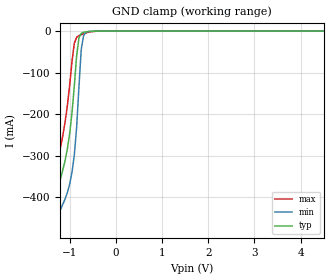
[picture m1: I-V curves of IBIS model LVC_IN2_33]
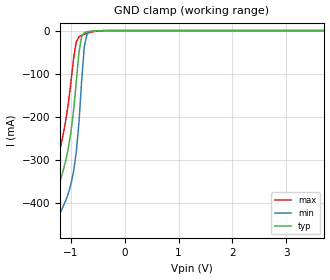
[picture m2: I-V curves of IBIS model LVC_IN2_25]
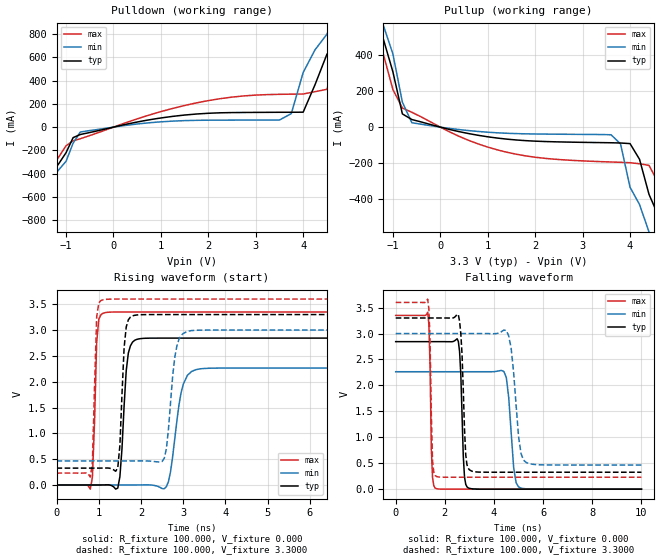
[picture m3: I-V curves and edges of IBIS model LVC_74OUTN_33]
| Philips Semiconductors Inc.
| Logic Products Group
| IBIS model of 74LVC74A
| DUAL D-TYPE FLIP-FLOP WITH SET AND RESET; POSITIVE-EDGE TRIGGER
|[Packages]:
|[Package1]: SO 14-pin (D) Package ;
|[Package2]: SSOP 14-Pin Packages ;
|[Package3]: TSSOP 14-pin (PW) Package ;
[IBIS Ver]   3.2
[File Name]   lvc74a.ibs
[File Rev]   1.3
[Date]   26-Nov-2002
[Source]   File created from simulations by LPG
   Philips Semiconductors Nijmegen
[Notes]   V1.3   Ibis model.
| Remark:
| The Power Clamp curves have been omitted since there is no power clamp diode.
| Revision History
| Version Date   Author/ Description
|   Editor
| 1.0   1999   Initial Version
| 1.1   October, 2001 RM   Revised for Ibis 3.2:
|   Model Spec and Model Selector added
| 1.2   November 2001 RM   Monotonous Curves
| 1.3   November 2002 RM   Revised: Power Clamp curves omitted, constant
|   end points for Ground Clamp and V/t curves.
[Disclaimer]
   (C) Copyright 2002 Philips Semiconductors
   All rights reserved
   Philips Semiconductors warrants and represents that the IBIS model
   identified herein is owned by Philips Semiconductors (PHILIPS). The
   model provided is not warranted as fully representing all of the
   operating characteristics and specifications of the semiconductor
   products to which the model relates.  Moreover, unless there is a
   signed, written agreement to the contrary, this IBIS model is
   furnished on an "as is" basis without support or warranty of any
   kind, either expressed or implied, regarding the use thereof, and
   PHILIPS specifically disclaims all implied warranties of
   merchantability and fitness of the model for any purpose.
   PHILIPS does not assume any liability arising out of the application
   or use of this IBIS model including infringement of patents and
   copyrights, nor does PHILIPS convey any license under its patents and
   copyrights or the rights of others.
   PHILIPS provides IBIS models as a service to our customers. You and
   your company shall not distribute, convey, sell, or give these models
   to anyone else without receiving prior written permission from
   PHILIPS.
   PHILIPS reserves the right to make changes without notice to these
   IBIS models to improve reliability, function, or design.
   Please be aware that your receipt and subsequent use of the IBIS
   information provided shall serve as acceptance of the terms and
   conditions of this agreement.  If you do not accept these terms,
   you should return or destroy the IBIS models and any other
   accompanying information immediately.
| to specify a consistent format that can be parsed by software, allowing
| simulation vendors to derive models compatible with their own products.
| One goal of this template is to represent the current state of IBIS data,
| while allowing a growth path to more complex models / methods (when deemed
| appropriate).  This would be accomplished by a revision of the base
| template, and possibly the addition of new keywords or categories.
| Another goal of this template is to ensure that it is simple enough for
| semiconductor vendors and customers to use and modify, while ensuring that
| it is rigid enough for simulation vendors to write reliable parsers.
| Finally, this template is meant to contain a complete description of the I/O
| elements on an entire component.  Consequently, several models will need to
| be defined in each file, as well as a table that equates the appropriate
| buffer to the correct pin and signal name.
| Version 3.2 of this electronic template was finalized by an industry-wide
| group of experts representing various companies and interests.  Regular
| "EIA IBIS Open Forum" meetings were held to accomplish this task.
| Commitment to Backward Compatibility.  Version 1.0 is the first valid IBIS
| ASCII file format.  It represents the minimum amount of I/O buffer
| information required to create an accurate IBIS model of common CMOS and
| bipolar I/O structures.  Future revisions of the ASCII file will add items
| considered to be "enhancements" to Version 1.0 to allow accurate modeling
| of new, or other I/O buffer structures.  Consequently, all future revisions
| will be considered supersets of Version 1.0, allowing backward
| compatibility.  In addition, as modeling platforms develop support for
| revisions of the IBIS ASCII template, all previous revisions of the template
| must also be supported.
| Version 1.1 update.  The file "ver1_1.ibs" is conceptually the same as the
| 1.0 version of the IBIS ASCII format (ver1_0.ibs).  However, various
| comments have been added for further clarification.
| Version 2.0 update.  The file "ver2_0.ibs" maintains backward compatibility
| with Versions 1.0 and 1.1.  All new keywords and elements added in Version
| 2.0 are optional.  A complete list of changes to the specification is in the
| IBIS Version 2.0 Release Notes document ("ver2_0.rn").
| Version 2.1 update.  The file "ver2_1.ibs" contains clarification text
| changes, corrections, and two additional waveform parameters beyond
| Version 2.0.
| Version 3.0 update.  The file "ver3_0.ibs" adds a number of new keywords
| and functionality.  A complete list of functions can be found on eda.org
| under /pub/ibis/birds/birddir.txt showing the approved Buffer Issue
| Resolution Documents (BIRDs) that have been approved for Version 3.0.
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[Component]   74LVC74A_1
[Manufacturer]   Philips Semiconductors Inc.
[Package]
|   typ   min   max
R_pkg   4.54E-02   4.18E-02   5.01E-02
L_pkg   2.31E-09   1.63E-09   3.26E-09
C_pkg   0.565E-12  0.437E-12  0.736E-12
[Pin] signal_name   model_name   R_pin   L_pin   C_pin
   1   1RD#   lvc_in2 4.18E-02 3.26E-09 0.675E-12
   2   1D   lvc_in2 5.01E-02 2.30E-09 0.574E-12
   3   1CP   lvc_in2 4.52E-02 1.71E-09 0.467E-12
   4   1SD#   lvc_in2 4.38E-02 1.63E-09 0.437E-12
   5   1Q   lvc_74outn 4.52E-02 1.71E-09 0.465E-12
   6   1QBAR#   lvc_74outi 5.01E-02 2.30E-09 0.573E-12
   7   GND   GND 4.18E-02 3.26E-09 0.736E-12
   8   2QBAR#   lvc_74outi 4.18E-02 3.26E-09 0.736E-12
   9   2Q   lvc_74outn 5.01E-02 2.30E-09 0.573E-12
   10   2SD#   lvc_in2 4.52E-02 1.71E-09 0.465E-12
   11   2CP   lvc_in2 4.38E-02 1.63E-09 0.437E-12
   12   2D   lvc_in2 4.52E-02 1.71E-09 0.467E-12
   13   2RD#   lvc_in2 5.01E-02 2.30E-09 0.574E-12
   14   VCC   POWER 4.18E-02 3.26E-09 0.736E-12
|   Info for  SSOP 14-Pin Packages
[Component]   74LVC74A_2
[Manufacturer]   Philips Semiconductors Inc.
[Package]
|   typ   min   max
R_pkg   18.10E-03   15.70E-03   19.10E-03
L_pkg   2.12E-09   1.76E-09   2.65E-09
C_pkg   0.59E-12   0.55E-12   0.64E-12
[Pin] signal_name   model_name   R_pin   L_pin   C_pin
   1   1RD#   lvc_in2 19.10E-03 2.65E-09 0.58E-12
   2   1D   lvc_in2 17.70E-03 2.07E-09 0.64E-12
   3   1CP   lvc_in2 18.70E-03 1.82E-09 0.57E-12
   4   1SD#   lvc_in2 15.70E-03 1.76E-09 0.55E-12
   5   1Q   lvc_74outn 18.70E-03 1.82E-09 0.57E-12
   6   1QBAR#   lvc_74outi 17.70E-03 2.07E-09 0.63E-12
   7   GND   GND 19.10E-03 2.65E-09 0.60E-12
   8   2QBAR#   lvc_74outi 19.10E-03 2.65E-09 0.60E-12
   9   2Q   lvc_74outn 17.80E-03 2.07E-09 0.64E-12
   10   2SD#   lvc_in2 18.70E-03 1.82E-09 0.57E-12
   11   2CP   lvc_in2 15.70E-03 1.76E-09 0.55E-12
   12   2D   lvc_in2 18.70E-03 1.82E-09 0.57E-12
   13   2RD#   lvc_in2 17.80E-03 2.07E-09 0.64E-12
   14   VCC   POWER 19.10E-03 2.65E-09 0.60E-12
|   Info for  TSSOP 14-pin (PW) Package
[Component]   74LVC74A_3
[Manufacturer]   Philips Semiconductors Inc.
[Package]
|   typ   min   max
R_pkg   3.44E-02   2.80E-02   4.33E-02
L_pkg   1.83E-09   1.36E-09   2.32E-09
C_pkg   0.380E-12  0.302E-12  0.442E-12
[Pin] signal_name   model_name   R_pin   L_pin   C_pin
   1   1RD#   lvc_in2 3.46E-02 2.32E-09 0.423E-12
   2   1D   lvc_in2 4.33E-02 2.04E-09 0.441E-12
   3   1CP   lvc_in2 2.80E-02 1.36E-09 0.307E-12
   4   1SD#   lvc_in2 2.88E-02 1.38E-09 0.302E-12
   5   1Q   lvc_74outn 2.80E-02 1.36E-09 0.308E-12
   6   1QBAR#   lvc_74outi 4.33E-02 2.04E-09 0.441E-12
   7   GND   GND 3.46E-02 2.32E-09 0.433E-12
   8   2QBAR#   lvc_74outi 3.46E-02 2.32E-09 0.433E-12
   9   2Q   lvc_74outn 4.33E-02 2.04E-09 0.441E-12
   10   2SD#   lvc_in2 2.80E-02 1.36E-09 0.308E-12
   11   2CP   lvc_in2 2.88E-02 1.38E-09 0.302E-12
   12   2D   lvc_in2 2.80E-02 1.36E-09 0.308E-12
   13   2RD#   lvc_in2 4.33E-02 2.04E-09 0.442E-12
   14   VCC   POWER 3.46E-02 2.31E-09 0.433E-12
[Model Selector]   lvc_in2
| Remark: If your software does not support the Model Selector
|   Please comment out the lines of the Model Selector, which
|   contain the name of the Model, except the one you want to use.
LVC_IN2_33   3.3V-Vcc input model
LVC_IN2_25   2.5V-Vcc input model
[Model Selector]   lvc_74outn
| Remark: If your software does not support the Model Selector
|   Please comment out the lines of the Model Selector, which
|   contain the name of the Model, except the one you want to use.
LVC_74OUTN_33   3.3V-Vcc non-inverting output model
LVC_74OUTN_25   2.5V-Vcc non-inverting output model
[Model Selector]   lvc_74outi
| Remark: If your software does not support the Model Selector
|   Please comment out the lines of the Model Selector, which
|   contain the name of the Model, except the one you want to use.
LVC_74OUTI_33   3.3V-Vcc inverting output model
LVC_74OUTI_25   2.5V-Vcc inverting output model
| Models and submodels in the file (6): LVC_IN2_33 (Input), LVC_IN2_25 (Input), LVC_74OUTN_33 (Output), LVC_74OUTN_25 (Output), LVC_74OUTI_33 (Output), LVC_74OUTI_25 (Output)
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|   Model LVC_IN2_33
[Model]   LVC_IN2_33
Model_type   Input
Vinl =   0.8000V
Vinh =   2.0000V
C_comp   2.78pF   1.99pF   3.72pF
[Model Spec]
| Note: The input and output voltage ratings may be exceeded if the input and
|   output current ratings are observed (please refer to the data sheet)
|   Subparameter   typ   min   max
| Thresholds
Vinh   2.0   NA   NA
Vinl   0.8   NA   NA
| Overshoot
S_overshoot_high   6.5   6.5   6.5   | Static overshoot
S_overshoot_low   -0.5   -0.5   -0.5
D_overshoot_high   7.2   7.2   7.2   | Dynamic overshoot
D_overshoot_low   -0.95   -0.9   -1.0
D_overshoot_time   3n   3n   3n
|Ambient temperature:   25.0000   85.0000   -40.0000
[Temperature Range]   40.0000   100.0000   -25.0000
[Voltage Range]   3.3000V   3.0000V   3.6000V
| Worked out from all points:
|   GND clamp passes 1 mA (typ) near -0.57 V on its own axis
|Process Range   nominal   slow   fast
[GND_clamp]
| voltage   I(typ)   I(min)   I(max)
-5.5V     -4.567A    -4.624A    -4.51A
-1.45V    -555.2mA   -621.5mA   -488.4mA
-1.35V    -461.8mA   -528.7mA   -394.3mA
-1.3V     -417.5mA   -485mA     -349.4mA
-1.1V     -312.4mA   -404.8mA   -219.8mA
-950mV    -197.3mA   -340.4mA   -73.13mA
-900mV    -132mA     -298.5mA   -29.44mA
-850mV    -59.79mA   -233mA     -14.94mA
-800mV    -16.87mA   -135mA     -10.93mA
-750mV    -5.479mA   -44.49mA   -8.487mA
-700mV    -2.88mA    -11.01mA   -6.407mA
5.5V      1.567nA    9.324nA    202.5pA
|   Model LVC_IN2_25
[Model]   LVC_IN2_25
Model_type   Input
Vinl =   0.7000V
Vinh =   1.7000V
C_comp   2.84pF   2.10pF   3.71pF
[Model Spec]
| Note: The input and output voltage ratings may be exceeded if the input and
|   output current ratings are observed (please refer to the data sheet)
|   Subparameter   typ   min   max
| Thresholds
Vinh   1.7   NA   NA
Vinl   0.7   NA   NA
| Overshoot
S_overshoot_high   6.5   6.5   6.5   | Static overshoot
S_overshoot_low   -0.5   -0.5   -0.5
D_overshoot_high   7.2   7.2   7.2   | Dynamic overshoot
D_overshoot_low   -0.95   -0.9   -1.0
D_overshoot_time   3n   3n   3n
|Ambient temperature:   25.0000   85.0000   -40.0000
[Temperature Range]   35.0000   95.0000   -30.0000
[Voltage Range]   2.5000V   2.3000V   2.7000V
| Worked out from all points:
|   GND clamp passes 1 mA (typ) near -0.57 V on its own axis
|Process Range   nominal   slow   fast
[GND_clamp]
| voltage   I(typ)   I(min)   I(max)
-5.5V     -4.558A    -4.615A    -4.502A
-1.45V    -549mA     -615mA     -482.5mA
-1.35V    -455.6mA   -522.2mA   -388.4mA
-1.3V     -411.3mA   -478.6mA   -343.5mA
-1.1V     -304mA     -396mA     -212mA
-950mV    -185.1mA   -326.6mA   -65.02mA
-900mV    -119.1mA   -281.8mA   -26.08mA
-850mV    -50.24mA   -213.2mA   -14.46mA
-800mV    -13.81mA   -116mA     -10.88mA
-750mV    -4.865mA   -35.92mA   -8.446mA
-700mV    -2.732mA   -8.828mA   -6.333mA
5.5V      922.9pA    6.4nA      86.94pA
|   Model LVC_74OUTN_33
[Model]   LVC_74OUTN_33
Model_type   Output
Polarity   Non-Inverting
Vmeas =  1.5000V
Cref  = 50.0000pF
Rref  =  0.5000k
Vref  =  0.000V
C_comp   3.12pF   2.70pF   3.60pF
[Model Spec]
| Note: The input and output voltage ratings may be exceeded if the input and
|   output current ratings are observed (please refer to the data sheet)
|   Subparameter   typ   min   max
| Timing Thresholds
Vmeas   1.5   1.5   1.5
|Ambient temperature:   25.0000   85.0000   -40.0000
[Temperature Range]   40.0000   100.0000   -25.0000
[Voltage Range]   3.3000V   3.0000V   3.6000V
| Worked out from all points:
|   slope of the pulldown table from 0 to 0.495 V, typ, clamps not added: 11.4 ohm
|   slope of the pullup table from 0 to 0.495 V, typ, clamps not added: 16.3 ohm
|   rising waveform, R_fixture 100.000, V_fixture 0.000: 20-80 % time 122ps typ, 224ps min, 73.5ps max; typ from 0 V to 2.84 V
|   rising waveform, R_fixture 100.000, V_fixture 3.3000: 20-80 % time 97.8ps typ, 168ps min, 72.3ps max; typ from 0.327 V to 3.3 V
|   falling waveform, R_fixture 100.000, V_fixture 0.000: 20-80 % time 116ps typ, 207ps min, 79.5ps max; typ from 2.84 V to 0 V
|   falling waveform, R_fixture 100.000, V_fixture 3.3000: 20-80 % time 137ps typ, 267ps min, 86.9ps max; typ from 3.3 V to 0.327 V
|Process Range   nominal   slow   fast
[Pulldown]
| voltage   I(typ)   I(min)   I(max)
-5.5V     -4.549A    -4.579A    -4.522A
-1.9V     -966mA     -1.008A    -917mA
-1.75V    -820.1mA   -862.9mA   -770.2mA
-1.3V     -396.9mA   -441.3mA   -346.4mA
-700mV    -63.6mA    -42.24mA   -99.98mA
3.5V      127.9mA    61.26mA    282.4mA
3.75V     128.1mA    116.3mA    283.9mA
4V        128.6mA    470mA      285mA
4.5V      626.1mA    799.2mA    325.5mA
4.75V     782.1mA    1.022A     640.2mA
5.25V     1.248A     1.522A     1.043A
11V       6.834A     7.16A      6.528A
[Pullup]
| voltage   I(typ)   I(min)   I(max)
-8V       7.11A      7.148A     7.074A
-1.6V     743.7mA    798mA      683.2mA
-1.2V     489.6mA    565.9mA    405.1mA
-800mV    73.9mA     139.3mA    106.8mA
-600mV    42.4mA     24.62mA    82.79mA
1.2V      -60.89mA   -31.54mA   -126.5mA
3.6V      -87.04mA   -42.47mA   -194.3mA
3.8V      -88.38mA   -93.57mA   -196mA
4V        -91.76mA   -334.9mA   -198.2mA
4.4V      -374.8mA   -584.4mA   -213.2mA
5V        -890.4mA   -1.179A    -648.8mA
9.1V      -5.171A    -5.392A    -5.05A
[Ramp]
| variable   typ   min   max
dV/dt_r   1.706V/121.822ps   1.359V/224.056ps   2.010V/73.473ps
dV/dt_f   1.784V/137.324ps   1.521V/266.558ps   2.022V/86.926ps
R_load = 100.000
[Rising Waveform]
R_fixture   = 100.000
V_fixture   = 0.000
V_fixture_min = 0.000
V_fixture_max = 0.000
| time   V(typ)   V(min)   V(max)
0s        116.3pV    3.037nV    937.7pV
800ps     -40.85uV   4.954uV    -81.09mV
950ps     -102.5uV   -6.457uV   2.752V
1.1ns     657.9uV    -12.32uV   3.324V
1.45ns    -61.02mV   -28.48uV   3.349V
1.7ns     2.555V     -107.7uV   3.35V
1.9ns     2.819V     302.3uV    3.35V
2.6ns     2.844V     -33.78mV   3.35V
3.3ns     2.844V     2.233V     3.35V
10ns      2.844V     2.264V     3.35V
[Rising Waveform]
R_fixture   = 100.000
V_fixture   = 3.3000
V_fixture_min = 3.0000
V_fixture_max = 3.6000
| time   V(typ)   V(min)   V(max)
0s        326.6mV    465.6mV    230.2mV
800ps     326.6mV    465.6mV    153.2mV
950ps     326.5mV    465.6mV    3.25V
1.05ns    326.8mV    465.6mV    3.571V
1.45ns    334.4mV    465.7mV    3.6V
1.6ns     2.661V     465.7mV    3.6V
1.8ns     3.275V     465.9mV    3.6V
2.55ns    3.3V       518mV      3.6V
3.1ns     3.3V       2.975V     3.6V
10ns      3.3V       3V         3.6V
[Falling Waveform]
R_fixture   = 100.000
V_fixture   = 0.000
V_fixture_min = 0.000
V_fixture_max = 0.000
| time   V(typ)   V(min)   V(max)
0s        2.844V     2.264V     3.35V
1.3ns     2.844V     2.264V     3.411V
1.45ns    2.844V     2.264V     771.9mV
1.6ns     2.844V     2.264V     23.68mV
2.55ns    2.848V     2.264V     196.4nV
2.8ns     234.5mV    2.264V     13.96nV
2.95ns    24.91mV    2.264V     7.081nV
4.4ns     866.6nV    2.27V      1.519nV
5ns       14.77nV    43.65mV    1.549nV
10ns      150.4pV    4.487nV    1.479nV
[Falling Waveform]
R_fixture   = 100.000
V_fixture   = 3.3000
V_fixture_min = 3.0000
V_fixture_max = 3.6000
| time   V(typ)   V(min)   V(max)
0s        3.3V       3V         3.6V
1.3ns     3.3V       3V         3.665V
1.4ns     3.3V       3V         2.826V
1.5ns     3.3V       3V         538.5mV
1.65ns    3.3V       3V         247.1mV
2.55ns    3.36V      3V         230.2mV
3ns       372.7mV    3V         230.2mV
4.6ns     326.6mV    2.953V     230.2mV
5.3ns     326.6mV    517mV      230.2mV
10ns      326.6mV    465.6mV    230.2mV
